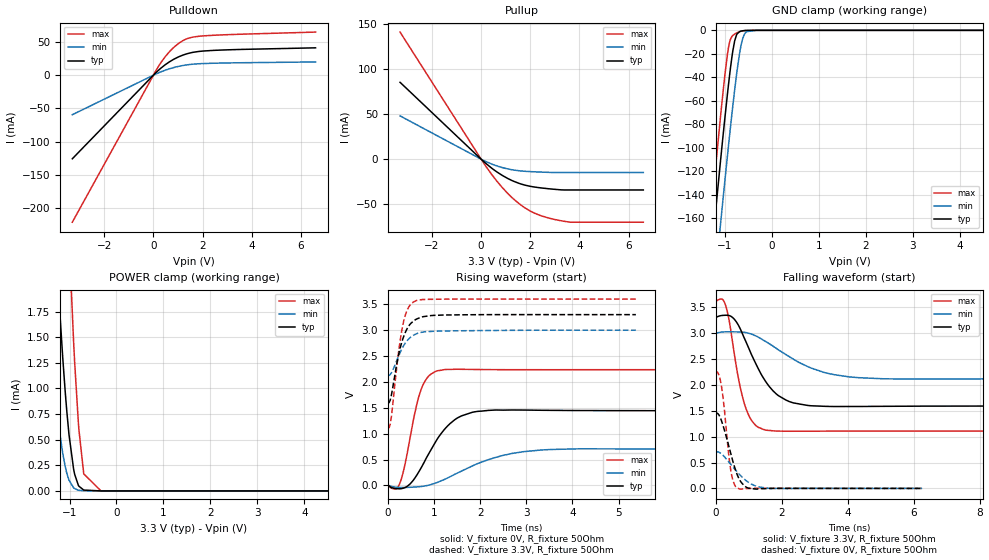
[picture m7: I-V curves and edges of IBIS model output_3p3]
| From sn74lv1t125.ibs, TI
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|   output_3p3 Model
[Model]   output_3p3
Model_type   3-state
Polarity   Non-Inverting
Vmeas = 1.65
Vref = 0
Cref = 50pF
Rref = 150
|   typ   min   max
|   (nom PVT)   (fast PVT)   (slow PVT)
C_comp   3.211e-12   3.100e-12   3.305e-12
| Where nom  PVT is Nominal Process, 3.3V, 40C
|   Fast PVT is Strong Process,  3.6V, -40C
|   Slow PVT is Weak Process,   3V, 140C
[Voltage Range]   3.3   3   3.6
|Junction Temperature
[Temperature Range]   40   140   -40
[Pullup Reference]   3.3   3   3.6
[Pulldown Reference]   0   0   0
[Power Clamp Reference]   3.3   3   3.6
[GND Clamp Reference]   0   0   0
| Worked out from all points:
|   slope of the pulldown table from 0 to 0.495 V, typ, clamps not added: 30.8 ohm
|   slope of the pullup table from 0 to 0.495 V, typ, clamps not added: 44.1 ohm
|   GND clamp passes 1 mA (typ) near -0.68 V on its own axis
|   POWER clamp passes 1 mA (typ) near -1.10 V on its own axis
|   falling waveform, V_fixture 3.3V, R_fixture 50Ohm: 20-80 % time 841ps typ, 1.48ns min, 438ps max; typ from 3.3 V to 1.59 V
|   rising waveform, V_fixture 0V, R_fixture 50Ohm: 20-80 % time 615ps typ, 1.13ns min, 315ps max; typ from 0 V to 1.45 V
|   rising waveform, V_fixture 3.3V, R_fixture 50Ohm: 20-80 % time 266ps typ, 306ps min, 214ps max; typ from 1.59 V to 3.3 V
|   falling waveform, V_fixture 0V, R_fixture 50Ohm: 20-80 % time 388ps typ, 609ps min, 219ps max; typ from 1.45 V to 0 V
[Pulldown]
|   Voltage   I(typ)   I(min)   I(max)
-3.3V     -125.5mA   -59.36mA   -220.8mA
156mV     5.69mA     2.699mA    10.19mA
458.4mV   15.09mA    7.21mA     26.68mA
634.8mV   19.65mA    9.42mA     34.51mA
1.006V    27.21mA    13.11mA    47.19mA
1.242V    30.72mA    14.81mA    52.73mA
1.445V    32.98mA    15.9mA     55.78mA
1.971V    36.11mA    17.41mA    58.87mA
3.231V    38.35mA    18.52mA    61.15mA
6.6V      41.11mA    19.9mA     64.75mA
[GND Clamp]
|   Voltage   I(typ)   I(min)   I(max)
-3.3V     -1.077A    -1.114A    -1.054A
-1.65V    -345.8mA   -396.9mA   -311.8mA
-1.228V   -165.4mA   -219.1mA   -128mA
-1.097V   -111.7mA   -165.6mA   -73.91mA
-999.9mV  -73.54mA   -127mA     -37mA
-924mV    -45.58mA   -97.6mA    -14.22mA
-884.4mV  -32.26mA   -82.72mA   -7.637mA
-795.3mV  -9.152mA   -51.02mA   -3.205mA
-687mV    -1.037mA   -18.94mA   -1.1mA
-591mV    -239.6uA   -3.513mA   -263.8uA
-330mV    -1.802uA   -6.695uA   -641.1nA
6.6V      0A         0A         0A
[Pullup]
|   Voltage   I(typ)   I(min)   I(max)
-3.3V     85.01mA    47.89mA    140.5mA
201mV     -4.872mA   -2.673mA   -8.194mA
481.8mV   -10.98mA   -5.876mA   -18.76mA
872.4mV   -18.12mA   -9.342mA   -31.73mA
1.251V    -23.54mA   -11.65mA   -42.32mA
1.549V    -26.76mA   -12.8mA    -49.25mA
1.967V    -29.8mA    -13.66mA   -56.83mA
2.395V    -31.61mA   -14.2mA    -62.11mA
3.386V    -34.02mA   -14.71mA   -68.67mA
3.633V    -34.02mA   -14.71mA   -69.64mA
6.6V      -34.02mA   -14.71mA   -69.64mA
[POWER Clamp]
|   Voltage   I(typ)   I(min)   I(max)
-3.3V     35.19mA    19.48mA    61.17mA
-1.529V   4.782mA    2.129mA    11.02mA
-1.36V    3.044mA    1.206mA    7.728mA
-1.29V    2.417mA    885.6uA    6.496mA
-1.205V   1.728mA    553.7uA    5.101mA
-1.092V   966.5uA    237.2uA    3.474mA
-1.011V   547.2uA    104.5uA    2.471mA
-913.2mV  211.9uA    30.43uA    1.453mA
-811.8mV  54.34uA    7.094uA    664.9uA
-697.2mV  8.348uA    1.28uA     166.3uA
-330mV    29.35nA    17.89nA    239nA
6.6V      0A         0A         0A
[Ramp]
R_load = 50
|   typ   min   max
dV/dt_r   0.867306/6.14864e-10   0.420514/1.12614e-09   1.34175/3.15228e-10
dV/dt_f   1.0258/8.40264e-10   0.528639/1.46179e-09   1.49523/4.384e-10
[Falling Waveform]
V_fixture = 3.3V
V_fixture_min = 3V
V_fixture_max = 3.6V
R_fixture = 50Ohm
|   Time   V(typ)   V(min)   V(max)
0s        3.3V       3V         3.6V
200ps     3.34V      3.02V      3.655V
325ps     3.344V     3.024V     3.484V
700ps     3.138V     3.022V     2.092V
925ps     2.822V     3.008V     1.531V
1.15ns    2.496V     2.963V     1.262V
1.425ns   2.154V     2.87V      1.144V
2.225ns   1.678V     2.546V     1.104V
4.05ns    1.582V     2.153V     1.107V
11.88ns   1.59V      2.119V     1.108V
[Rising Waveform]
V_fixture = 0V
V_fixture_min = 0V
V_fixture_max = 0V
R_fixture = 50Ohm
|   Time   V(typ)   V(min)   V(max)
0s        458.5pV    4.244nV    826.8pV
250ps     -63.99mV   -37.99mV   24.69mV
475ps     24.78mV    -35.09mV   892.9mV
700ps     309mV      -21.82mV   1.803V
875ps     597.1mV    4.557mV    2.105V
1.075ns   904.6mV    60.68mV    2.215V
1.525ns   1.313V     247.9mV    2.245V
2.175ns   1.45V      497.8mV    2.238V
3.55ns    1.451V     695.3mV    2.236V
9.2ns     1.446V     700.8mV    2.236V
[Rising Waveform]
V_fixture = 3.3V
V_fixture_min = 3V
V_fixture_max = 3.6V
R_fixture = 50Ohm
|   Time   V(typ)   V(min)   V(max)
0s        1.59V      2.119V     1.108V
50ps      1.647V     2.143V     1.181V
75ps      1.743V     2.174V     1.321V
225ps     2.495V     2.484V     2.528V
325ps     2.835V     2.676V     3.106V
425ps     3.041V     2.804V     3.402V
575ps     3.189V     2.911V     3.554V
775ps     3.262V     2.966V     3.593V
1.225ns   3.293V     2.984V     3.599V
5.375ns   3.3V       3V         3.6V
[Falling Waveform]
V_fixture = 0V
V_fixture_min = 0V
V_fixture_max = 0V
R_fixture = 50Ohm
|   Time   V(typ)   V(min)   V(max)
0s        1.446V     700.9mV    2.236V
75ps      1.439V     704mV      2.225V
150ps     1.353V     680.2mV    2.067V
225ps     1.213V     638.6mV    1.75V
450ps     694.2mV    469.8mV    385.3mV
525ps     514.6mV    412.1mV    149.3mV
650ps     270.9mV    319.5mV    8.038mV
950ps     15.38mV    136.7mV    -2.306mV
1.55ns    -3.486mV   6.528mV    1.018mV
6.25ns    -19.11uV   -123.4uV   2.199uV
